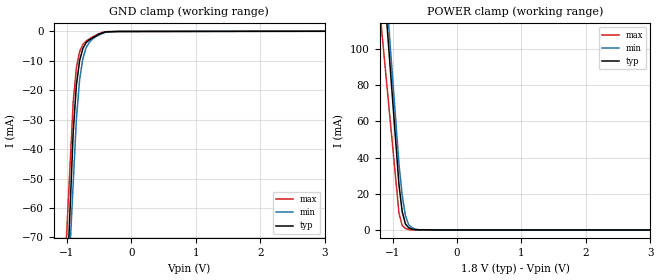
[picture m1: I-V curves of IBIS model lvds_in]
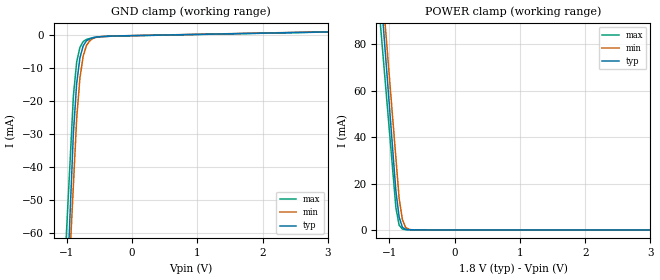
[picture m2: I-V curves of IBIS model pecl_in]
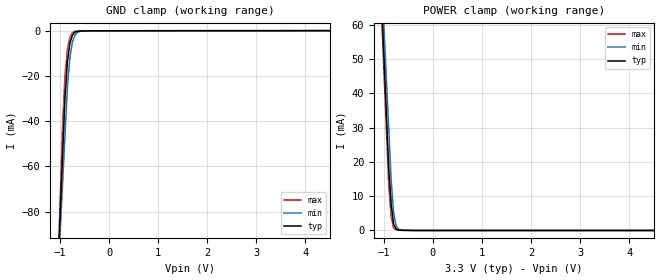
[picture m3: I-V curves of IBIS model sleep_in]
| Teraspeed Modeling Services.
| http://www.teraspeed.com
[IBIS Ver] 3.2
[File Name] dac3162.ibs
[File Rev] 3.0
[Date]   03-18-2011
[Notes]  Quality Check of this IBIS model: Model Passes IBIS Check. Model
   parses into ICX IS. Simulates with Hyperlynx.
   1. MIN TYP MAX information is based on Temperature and Voltage
   characteristics only.
   2. Package information extracted using Tektronix IConnect Software.
[Disclaimer]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
[Source]
| This model file was created by Teraspeed Consulting Group LLC
| (http://www.teraspeed.com/).
[Disclaimer]
| This product is designed as an aid for customers of Texas Instruments.
| No warranties, either expressed or implied, with respect to this third
| party software (if any) or with respect to its fitness for any
| particular purpose is claimed by Texas Instruments or the author. The
| software (if any) is provided solely on an "as is" basis. The entire
| risk as to its quality and performance is with the customer
[Copyright]
| (C) Copyright 2011 Texas Instruments Incorporated. All rights reserved.
| All other rights are reserved.
[Component] DAC3162
[Manufacturer] TI
[Package]
| variable   typ   min   max
R_pkg  1.000E-02   1.000E-02   1.000E-02
L_pkg  2.875E-09   2.600E-09   3.150E-09
C_pkg  6.167E-13   5.550E-13   6.783E-13
[Pin] signal_name  model_name  R_pin  L_pin C_pin
1   DACCLKP   pecl_in   1.000E-02 3.150E-09 6.783E-13
2   DACCLKN   pecl_in   1.000E-02 3.040E-09 6.537E-13
3   D11P   lvds_in   1.000E-02 2.930E-09 6.290E-13
4   D11N   lvds_in   1.000E-02 2.820E-09 6.043E-13
5   D10P   lvds_in   1.000E-02 2.710E-09 5.797E-13
6   D10N   lvds_in   1.000E-02 2.600E-09 5.550E-13
7   D9P   lvds_in   1.000E-02 2.600E-09 5.550E-13
8   D9N   lvds_in   1.000E-02 2.710E-09 5.797E-13
9   D8P   lvds_in   1.000E-02 2.820E-09 6.043E-13
10   D8N   lvds_in   1.000E-02 2.930E-09 6.290E-13
11   D7P   lvds_in   1.000E-02 3.040E-09 6.537E-13
12   D7N   lvds_in   1.000E-02 3.150E-09 6.783E-13
13   D6P   lvds_in   1.000E-02 3.150E-09 6.783E-13
14   D6N   lvds_in   1.000E-02 3.040E-09 6.537E-13
15   DVDD18   POWER   1.000E-02 2.930E-09 6.290E-13
16   D5P   lvds_in   1.000E-02 2.820E-09 6.043E-13
17   D5N   lvds_in   1.000E-02 2.710E-09 5.797E-13
18   VREF   term   1.000E-02 2.600E-09 5.550E-13
19   D4P   lvds_in   1.000E-02 2.600E-09 5.550E-13
20   D4N   lvds_in   1.000E-02 2.710E-09 5.797E-13
21   D3P   lvds_in   1.000E-02 2.820E-09 6.043E-13
22   D3N   lvds_in   1.000E-02 2.930E-09 6.290E-13
23   D2P   lvds_in   1.000E-02 3.040E-09 6.537E-13
24   D2N   lvds_in   1.000E-02 3.150E-09 6.783E-13
25   D1P   lvds_in   1.000E-02 3.150E-09 6.783E-13
26   D1N   lvds_in   1.000E-02 3.040E-09 6.537E-13
27   D0P   lvds_in   1.000E-02 2.930E-09 6.290E-13
28   D0N   lvds_in   1.000E-02 2.820E-09 6.043E-13
29   NC   NC   1.000E-02 2.710E-09 5.797E-13
30   NC   NC   1.000E-02 2.600E-09 5.550E-13
31   NC   NC   1.000E-02 2.600E-09 5.550E-13
32   NC   NC   1.000E-02 2.710E-09 5.797E-13
33   DVDD18   POWER   1.000E-02 2.820E-09 6.043E-13
34   SLEEPB   sleep_in  1.000E-02 2.930E-09 6.290E-13
35   ATEST   NC   1.000E-02 3.040E-09 6.537E-13
36   VFUSE   POWER   1.000E-02 3.150E-09 6.783E-13
37   IOUTBP   term   1.000E-02 3.150E-09 6.783E-13
38   IOUTBN   term   1.000E-02 3.040E-09 6.537E-13
39   GND   GND   1.000E-02 2.930E-09 6.290E-13
40   AVDD33   POWER   1.000E-02 2.820E-09 6.043E-13
41   DVDD18   POWER   1.000E-02 2.710E-09 5.797E-13
42   BIASJ   term   1.000E-02 2.600E-09 5.550E-13
43   AVDD33   POWER   1.000E-02 2.600E-09 5.550E-13
44   CLKVDD18  POWER   1.000E-02 2.710E-09 5.797E-13
45   AVDD33   POWER   1.000E-02 2.820E-09 6.043E-13
46   GND   GND   1.000E-02 2.930E-09 6.290E-13
47   IOUTAN   term   1.000E-02 3.040E-09 6.537E-13
48   IOUTAP   term   1.000E-02 3.150E-09 6.783E-13
[Diff Pin] inv_pin vdiff tdelay_typ tdelay_min tdelay_max
1   2   400mV   NA  NA  NA
3   4   150mV   NA  NA  NA
5   6   150mV   NA  NA  NA
7   8   150mV   NA  NA  NA
9   10  150mV   NA  NA  NA
11  12  150mV   NA  NA  NA
13  14  150mV   NA  NA  NA
16  17  150mV   NA  NA  NA
19  20  150mV   NA  NA  NA
21  22  150mV   NA  NA  NA
23  24  150mV   NA  NA  NA
25  26  150mV   NA  NA  NA
27  28  150mV   NA  NA  NA
[Series Pin Mapping] pin_2 model_name function_table_group
3   4   110ohm
5   6   110ohm
7   8   110ohm
9   10  110ohm
11  12  110ohm
13  14  110ohm
16  17  110ohm
19  20  110ohm
21  22  110ohm
23  24  110ohm
25  26  110ohm
27  28  110ohm
[Model]  110ohm
Model_type Series
C_comp   0   0   0
[Voltage Range]  1.80   1.70   1.90
[Temperature Range]   25   85   -40
[R series]   110   85   135
[Model]  term
Model_type Terminator
C_comp   0   0   0
[Voltage Range]  3.30  3.00  3.60
[Temperature Range]   25   85   -40
| Models and submodels in the file (5): lvds_in (Input), pecl_in (Input), sleep_in (Input), 110ohm (Series), term (Terminator)
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[Model] lvds_in
Model_type Input
Vinl = 1.12500V
Vinh = 1.27500V
C_comp 882.000fF 879.000fF 885.000fF
| variable typ   min   max
[Voltage Range] 1.80000V 1.70000V 1.90000V
[POWER Clamp Reference] 1.80000V 1.70000V 1.90000V
[GND Clamp Reference] 0.00000V 0.00000V 0.00000V
[Temperature Range]   25   85   -40
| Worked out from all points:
|   GND clamp passes 1 mA (typ) near -0.50 V on its own axis
|   POWER clamp passes 1 mA (typ) near -0.73 V on its own axis
[GND Clamp]
-1.8V     -516.4mA   -450.7mA   -422.4mA
-900mV    -34.53mA   -51.9mA    -24.17mA
-850mV    -18.27mA   -29.75mA   -12.3mA
-800mV    -9.904mA   -16.43mA   -6.903mA
-750mV    -5.838mA   -9.264mA   -4.466mA
-700mV    -3.875mA   -5.596mA   -3.283mA
-650mV    -2.888mA   -3.778mA   -2.59mA
-600mV    -2.244mA   -2.599mA   -1.898mA
-500mV    -957.3uA   -1.28mA    -772.7uA
-400mV    -203.4uA   -359.4uA   -116.6uA
-350mV    -165.3uA   -129.6uA   -92.98uA
3.6V      34.64uA    93.6uA     41.96uA
[POWER Clamp]
-1.8V     453.5mA    469.3mA    347.9mA
-1V       72.49mA    84.47mA    46.91mA
-900mV    24.87mA    36.36mA    9.282mA
-850mV    10.07mA    19.19mA    2.491mA
-800mV    3.31mA     7.858mA    827.6uA
-750mV    1.232mA    2.889mA    239.1uA
-700mV    479.2uA    1.326mA    35.61uA
-600mV    111.6uA    154.4uA    26.71uA
3.6V      0A         0A         0A
[Model] pecl_in
Model_type Input
Vinl = 400.000mV
Vinh = 1.00000V
C_comp 885.000fF 863.000fF 907.000fF
| variable typ   min   max
[Voltage Range] 1.80000V 1.70000V 1.90000V
[POWER Clamp Reference] 1.80000V 1.70000V 1.90000V
[GND Clamp Reference] 0.00000V 0.00000V 0.00000V
[Temperature Range]   25   85   -40
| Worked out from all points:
|   GND clamp passes 1 mA (typ) near -0.60 V on its own axis
|   POWER clamp passes 1 mA (typ) near -0.79 V on its own axis
[GND Clamp]
-1.8V     -461.7mA   -406.1mA   -369.2mA
-900mV    -29.73mA   -45.46mA   -18.51mA
-850mV    -14.79mA   -25.42mA   -8.318mA
-800mV    -7.02mA    -13.11mA   -3.88mA
-750mV    -3.412mA   -6.512mA   -2.125mA
-700mV    -1.892mA   -3.308mA   -1.472mA
-650mV    -1.305mA   -1.906mA   -1.2mA
-600mV    -985.7uA   -1.18mA    -928.5uA
-500mV    -673.3uA   -672.2uA   -695.2uA
3.6V      1.026mA    1.084mA    988.3uA
[POWER Clamp]
-1.8V     348.4mA    345.8mA    309.2mA
-1V       53.54mA    65.95mA    42.84mA
-900mV    16.68mA    30.97mA    9.541mA
-850mV    5.464mA    13.48mA    2.063mA
-800mV    1.156mA    4.432mA    378.8uA
-750mV    269.4uA    1.018mA    100.7uA
-700mV    89.55uA    281.3uA    88.83uA
-650mV    76.75uA    76.37uA    76.99uA
3.6V      0A         0A         0A
[Model] sleep_in
Model_type Input
Vinl = 800.000mV
Vinh = 2.00000V
C_comp 536.000fF 517.000fF 555.000fF
| variable typ   min   max
[Voltage Range] 3.30000V 3.00000V 3.60000V
[POWER Clamp Reference] 3.30000V 3.00000V 3.60000V
[GND Clamp Reference] 0.00000V 0.00000V 0.00000V
[Temperature Range]   25   85   -40
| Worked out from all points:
|   GND clamp passes 1 mA (typ) near -0.71 V on its own axis
|   POWER clamp passes 1 mA (typ) near -0.77 V on its own axis
[GND Clamp]
-3.3V     -1.297A    -1.083A    -1.631A
-950mV    -55.81mA   -67.94mA   -42.19mA
-900mV    -29.39mA   -46.34mA   -19.76mA
-850mV    -13.45mA   -24.74mA   -7.914mA
-800mV    -5.498mA   -11.75mA   -2.809mA
-750mV    -2.007mA   -5.127mA   -895.6uA
-700mV    -684.3uA   -2.081mA   -323.6uA
-650mV    -280uA     -853.7uA   -179.1uA
-600mV    -141.4uA   -311.8uA   -156.5uA
-500mV    -105.4uA   -75.74uA   -111.4uA
6.6V      42.24uA    53.3uA     37.93uA
[POWER Clamp]
-3.3V     814.2mA    756.5mA    823.8mA
-1.05V    67.84mA    75.1mA     64.03mA
-950mV    34.67mA    44.81mA    30.26mA
-900mV    18.09mA    29.67mA    13.38mA
-850mV    7.544mA    14.53mA    3.742mA
-800mV    1.804mA    5.144mA    735.4uA
-750mV    394.1uA    1.292mA    211.1uA
-700mV    143.7uA    391.2uA    117.2uA
-650mV    60.45uA    152.8uA    23.4uA
-450mV    23.25uA    0A         13.55uA
6.6V      0A         0A         0A
